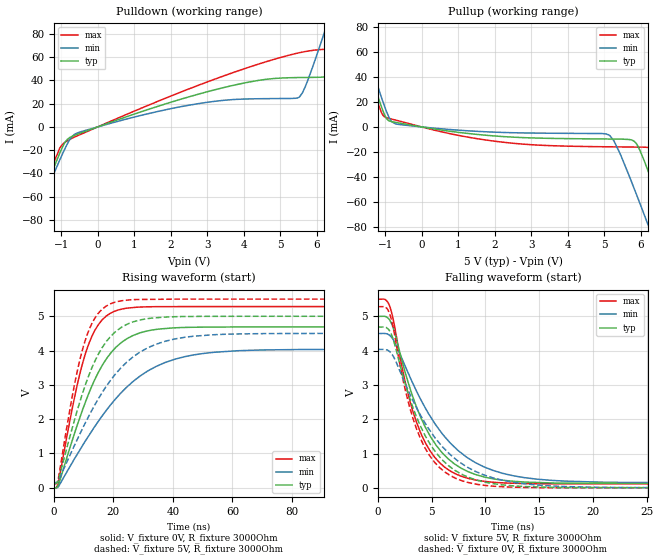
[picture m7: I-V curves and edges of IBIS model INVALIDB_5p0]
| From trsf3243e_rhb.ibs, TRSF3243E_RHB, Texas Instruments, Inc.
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[Model]   INVALIDB_5p0
Model_type   Output
Polarity   Inverting
Vmeas = 2.5
Vref = 2.5
Cref = 30pF
Rref = 0
|   typ   min   max
C_comp   1.08pF   1.06pF   1.09pF
|C_pullup   1.20pF   1.10pF   1.26pF
|C_pulldown   1.68pF   1.64pF   1.74pF
[Voltage Range]   5   4.5   5.5
[Temperature Range]   27   110   -40
[Pullup Reference]   5   4.5   5.5
[Pulldown Reference]   0   0   0
[Power Clamp Reference]   5   4.5   5.5
[GND Clamp Reference]   0   0   0
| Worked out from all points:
|   slope of the pulldown table from 0 to 0.75 V, typ, clamps not added: 90.1 ohm
|   slope of the pullup table from 0 to 0.75 V, typ, clamps not added: 223 ohm
|   falling waveform, V_fixture 5V, R_fixture 3000Ohm: 20-80 % time 3.79ns typ, 5.31ns min, 2.92ns max; typ from 5 V to 0.127 V
|   rising waveform, V_fixture 0V, R_fixture 3000Ohm: 20-80 % time 13ns typ, 21.8ns min, 8.43ns max; typ from 0 V to 4.69 V
|   rising waveform, V_fixture 5V, R_fixture 3000Ohm: 20-80 % time 11.6ns typ, 18.3ns min, 7.77ns max; typ from 0.127 V to 5 V
|   falling waveform, V_fixture 0V, R_fixture 3000Ohm: 20-80 % time 3.72ns typ, 5.06ns min, 2.9ns max; typ from 4.69 V to 0 V
[Pulldown]
|   Voltage   I(typ)   I(min)   I(max)
-5V       -356.4mA   -337.1mA   -375.9mA
-2.33V    -128.7mA   -126.8mA   -130.8mA
-1.64V    -70.76mA   -73.39mA   -68.44mA
-1.04V    -22.68mA   -28.58mA   -18.41mA
-620mV    -7.055mA   -6.072mA   -8.528mA
2.74V     27.99mA    19.93mA    35.55mA
5.5V      42.43mA    25.24mA    63.59mA
6.265V    43.14mA    86.4mA     66.81mA
6.88V     90.18mA    145.7mA    67.46mA
7.165V    117.5mA    173.5mA    69.53mA
7.48V     148.1mA    204.4mA    95.08mA
10V       396.9mA    453.5mA    342.4mA
[Pullup]
|   Voltage   I(typ)   I(min)   I(max)
-5V       396.7mA    403.7mA    391.7mA
-2.255V   125.3mA    132.9mA    119.7mA
-1.715V   72.75mA    80.64mA    67.02mA
-1.1V     16mA       23.53mA    11.43mA
-710mV    3.619mA    2.378mA    5.45mA
2.11V     -7.469mA   -4.305mA   -11.84mA
5.125V    -9.669mA   -6.386mA   -15.92mA
5.83V     -11.66mA   -50.12mA   -16.11mA
6.25V     -39.11mA   -82.19mA   -16.56mA
6.67V     -73.51mA   -114.8mA   -28.63mA
7.45V     -139.2mA   -175.9mA   -96.7mA
10V       -357mA     -377.6mA   -330.2mA
[Ramp]
R_load = 3000
|   typ   min   max
dV/dt_r   2.81344/1.30203e-08   2.42099/2.18395e-08   3.16968/8.43424e-09
dV/dt_f   2.92363/3.78816e-09   2.61073/5.31042e-09   3.23244/2.92395e-09
[Falling Waveform]
V_fixture = 5V
V_fixture_min = 4.5V
V_fixture_max = 5.5V
R_fixture = 3000Ohm
C_fixture = 0F
|   Time   V(typ)   V(min)   V(max)
0s        5V         4.5V       5.5V
1.146ns   4.868V     4.434V     5.258V
2.584ns   3.321V     3.516V     3.027V
3.266ns   2.641V     3.037V     2.219V
3.994ns   2.049V     2.57V      1.589V
5.257ns   1.317V     1.893V     900.9mV
7.122ns   696mV      1.188V     424.2mV
9.033ns   393.8mV    740.2mV    232.3mV
13.77ns   167.9mV    292mV      123.7mV
1us       127.3mV    148.8mV    112.6mV
[Rising Waveform]
V_fixture = 0V
V_fixture_min = 0V
V_fixture_max = 0V
R_fixture = 3000Ohm
C_fixture = 0F
|   Time   V(typ)   V(min)   V(max)
0s        -115.4nV   -132.9nV   -100.1nV
1.52ns    81.34mV    33.67mV    148.8mV
7.849ns   1.821V     974.1mV    2.992V
12.72ns   2.955V     1.648V     4.404V
19.2ns    3.938V     2.431V     5.096V
27.71ns   4.477V     3.173V     5.263V
37.42ns   4.642V     3.653V     5.281V
47.06ns   4.68V      3.875V     5.283V
82.38ns   4.689V     4.03V      5.283V
1us       4.689V     4.035V     5.283V
[Rising Waveform]
V_fixture = 5V
V_fixture_min = 4.5V
V_fixture_max = 5.5V
R_fixture = 3000Ohm
C_fixture = 0F
|   Time   V(typ)   V(min)   V(max)
0s        127.3mV    148.8mV    112.6mV
1.442ns   206.7mV    189.5mV    244.5mV
7.255ns   2.071V     1.295V     3.144V
9.203ns   2.633V     1.649V     3.891V
11.76ns   3.273V     2.09V      4.59V
17.66ns   4.267V     2.963V     5.3V
25.99ns   4.815V     3.771V     5.481V
40.63ns   4.987V     4.339V     5.5V
70.82ns   5V         4.495V     5.5V
1us       5V         4.5V       5.5V
[Falling Waveform]
|Gnd
V_fixture = 0V
V_fixture_min = 0V
V_fixture_max = 0V
R_fixture = 3000Ohm
C_fixture = 0F
|   Time   V(typ)   V(min)   V(max)
0s        4.689V     4.035V     5.283V
1.046ns   4.598V     3.988V     5.117V
2.584ns   2.992V     3.008V     2.805V
3.266ns   2.339V     2.541V     2.02V
3.994ns   1.777V     2.101V     1.412V
5.257ns   1.091V     1.484V     751mV
7.122ns   517mV      865mV      295.8mV
9.033ns   240.9mV    484mV      113.4mV
13.77ns   36.53mV    114.5mV    10.63mV
1us       -255.6nV   -189.9nV   -90.55nV
